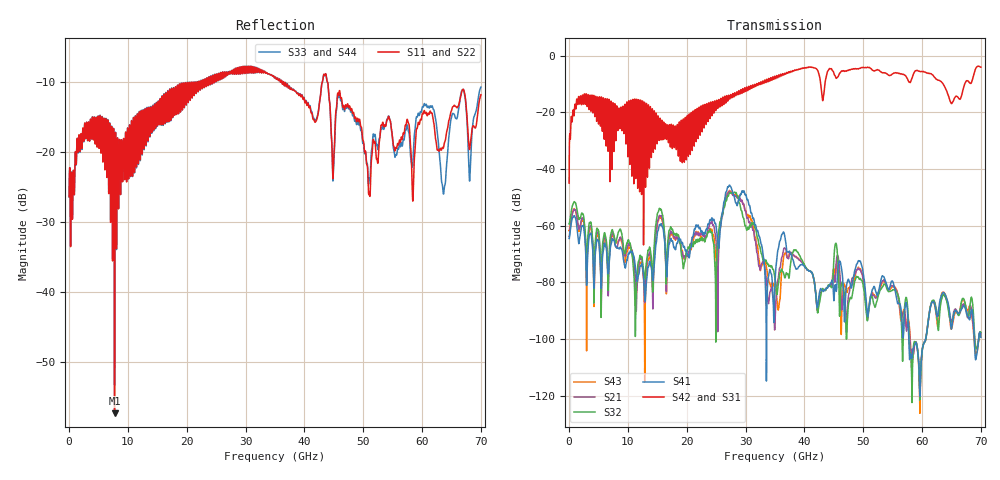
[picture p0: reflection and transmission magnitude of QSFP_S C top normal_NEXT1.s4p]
! AWR Design Environment (8415) Tue Jan 08 11:51:59 2019
! Document = 'QSFP Channel_S'
! nPorts: 4, nXvals: 7001
# HZ S DB R 50
!Freq DBS11 AngS11 DBS12 AngS12 DBS13 AngS13 DBS14 AngS14
!	DBS21 AngS21 DBS22 AngS22 DBS23 AngS23 DBS24 AngS24
!	DBS31 AngS31 DBS32 AngS32 DBS33 AngS33 DBS34 AngS34
!	DBS41 AngS41 DBS42 AngS42 DBS43 AngS43 DBS44 AngS44
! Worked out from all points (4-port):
!   7000 points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, 10 MHz to 70 GHz, reference 50 ohm
!   strongest paths, dB at 10 MHz, 17.51 GHz, 35.01 GHz, 52.51 GHz, 70 GHz:
!     S42: -45.0, -30.3, -7.3, -5.0, -4.0
!     S31: -44.9, -30.3, -7.3, -5.0, -4.0
!     S41: -64.5, -65.3, -80.1, -83.8, -99.4
!     S32: -59.4, -61.3, -78.8, -85.0, -97.7
!     S21: -63.8, -62.5, -94.4, -84.2, -98.1
!     S43: -61.8, -63.1, -82.6, -84.0, -98.9
!   lowest |S11| = -57.3 dB at 7.73 GHz (marker M1), VSWR 1.00, Z = 49.9 + j0.127 ohm
!   |S11| at or under -10 dB: start of sweep to 20.42 GHz; 36.48 GHz to 43.04 GHz (6.553 GHz wide, 16.5 % of centre); 43.96 GHz to end of sweep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
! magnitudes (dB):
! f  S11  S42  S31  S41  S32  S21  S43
! 10 MHz  -26.3  -45.0  -44.9  -64.5  -59.4  -63.8  -61.8
! 1.63 GHz  -18.3  -14.4  -14.4  -66.2  -57.6  -61.0  -61.8
! 7.73 GHz  -57.3  -18.1  -18.1  -65.8  -64.5  -64.9  -64.8
! 25.07 GHz  -9.1  -16.1  -16.0  -61.5  -73.6  -68.6  -81.2
! 27.25 GHz  -8.8  -15.0  -15.0  -45.7  -48.5  -47.9  -47.6
! 33.63 GHz  -8.6  -8.2  -8.2  -88.2  -73.3  -81.7  -75.6
! 70 GHz  -11.8  -4.0  -4.0  -99.4  -97.7  -98.1  -98.9
